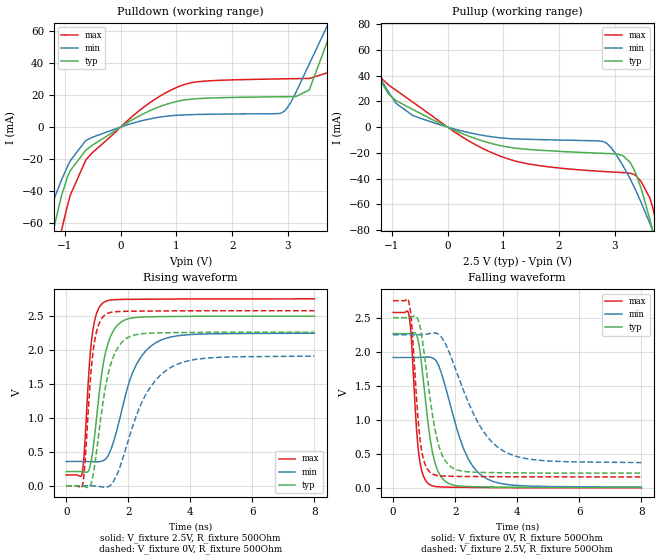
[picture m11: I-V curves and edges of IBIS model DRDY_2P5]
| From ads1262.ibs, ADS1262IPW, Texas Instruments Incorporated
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|   Model DRDY_2P5
[Model]   DRDY_2P5
Model_type   Output
Polarity   Non-Inverting
Enable   Active-Low
Vmeas = 1.25
Vref = 2.5
Cref = 15pF
Rref = 500
|   typ   min   max
|   (slow PVT)   (nom PVT)   (fast PVT)
C_comp   0.298p   0.274p   0.333p
|C_comp (ON state)   0.298p   0.282p   0.346p
|C_comp (OFF state)   0.298p   0.274p   0.333p
| Where   nom PVT is  Nominal Process, 2.5V, 27C
|   Fast PVT is Strong Process, 2.25V, -40C
|   Slow PVT is Weak Process, 2.75V, 125C
[Voltage Range]   2.5   2.25   2.75
[Temperature Range]   27   125   -40
[Pullup Reference]   2.5   2.25   2.75
[Pulldown Reference]   -0   -0   -0
[Power Clamp Reference]   2.5   2.25   2.75
[GND Clamp Reference]   -0   -0   -0
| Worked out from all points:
|   slope of the pulldown table from 0 to 0.375 V, typ, clamps not added: 48.4 ohm
|   slope of the pullup table from 0 to 0.375 V, typ, clamps not added: 54 ohm
|   falling waveform, V_fixture 0V, R_fixture 500Ohm: 20-80 % time 385ps typ, 813ps min, 219ps max; typ from 2.27 V to 0.006 V
|   rising waveform, V_fixture 2.5V, R_fixture 500Ohm: 20-80 % time 415ps typ, 791ps min, 236ps max; typ from 0.21 V to 2.5 V
|   rising waveform, V_fixture 0V, R_fixture 500Ohm: 20-80 % time 488ps typ, 1.03ns min, 262ps max; typ from 0 V to 2.26 V
|   falling waveform, V_fixture 2.5V, R_fixture 500Ohm: 20-80 % time 460ps typ, 1.13ns min, 251ps max; typ from 2.5 V to 0.216 V
[Pulldown]
|   Voltage   I(typ)   I(min)   I(max)
-2.5V     -315.8mA   -202.4mA   -454.5mA
-1.548V   -125.8mA   -82.52mA   -185.3mA
-1.315V   -83.24mA   -57.24mA   -122mA
-1.188V   -61.7mA    -44.53mA   -89.79mA
-1.06V    -42.72mA   -32.94mA   -64.38mA
-625mV    -14.46mA   -8.316mA   -20.61mA
950mV     15.58mA    7.244mA    24.01mA
2.877V    19mA       8.786mA    30.2mA
3.38V     23.15mA    39.24mA    30.47mA
3.703V    53.01mA    63.15mA    33.98mA
4.295V    106.5mA    98.71mA    106.7mA
4.992V    142.8mA    122.6mA    162.6mA
[Pullup]
|   Voltage   I(typ)   I(min)   I(max)
-2.5V     123.5mA    107.8mA    141.3mA
-1.87V    92.92mA    81.51mA    108.3mA
-1.645V   76.05mA    68.19mA    87.86mA
-1.06V    25.54mA    27.23mA    32.7mA
-625mV    13.67mA    9.005mA    19.41mA
950mV     -14.41mA   -8.361mA   -22.64mA
2.795V    -20.42mA   -11.34mA   -34.48mA
3.275V    -27.36mA   -40mA      -35.78mA
3.68V     -79.96mA   -80.27mA   -62.17mA
3.748V    -91.61mA   -87.8mA    -75.21mA
3.875V    -114.6mA   -102.5mA   -105.9mA
4.992V    -337mA     -247.2mA   -419.1mA
[Ramp]
R_load = 500
|   typ   min   max
dV/dt_r   1.3715/4.15054e-10   1.13197/7.90971e-10   1.55399/2.36049e-10
dV/dt_f   1.35577/3.84501e-10   1.14325/8.12774e-10   1.54566/2.19196e-10
[Falling Waveform]
V_fixture = 0V
V_fixture_min = 0V
V_fixture_max = 0V
R_fixture = 500Ohm
C_fixture = 0F
|   Time   V(typ)   V(min)   V(max)
0s        2.266V     1.915V     2.576V
504.3ps   2.265V     1.915V     2.549V
587.3ps   2.273V     1.915V     2.194V
817.8ps   2.142V     1.916V     535.8mV
943.9ps   1.704V     1.919V     217.6mV
1.18ns    768.1mV    1.919V     46.81mV
1.59ns    135.9mV    1.633V     12.85mV
2.278ns   22.4mV     565.7mV    7.372mV
2.883ns   14.06mV    171.6mV    5.396mV
8ns       5.923mV    9.605mV    126.9uV
[Rising Waveform]
V_fixture = 2.5V
V_fixture_min = 2.25V
V_fixture_max = 2.75V
R_fixture = 500Ohm
C_fixture = 0F
|   Time   V(typ)   V(min)   V(max)
0s        209.9mV    358.5mV    160mV
520.8ps   206.9mV    358.7mV    197.3mV
817.8ps   399.5mV    356mV      2.147V
943.9ps   855.7mV    353.9mV    2.485V
1.18ns    1.754V     369.1mV    2.69V
1.423ns   2.192V     517.1mV    2.732V
1.682ns   2.378V     907.7mV    2.74V
2.159ns   2.471V     1.687V     2.744V
2.883ns   2.488V     2.105V     2.746V
8ns       2.496V     2.245V     2.75V
[Rising Waveform]
V_fixture = 0V
V_fixture_min = 0V
V_fixture_max = 0V
R_fixture = 500Ohm
C_fixture = 0F
|   Time   V(typ)   V(min)   V(max)
0s        1.189nV    3.105nV    923.1pV
520.8ps   -2.675mV   352.2uV    4.909mV
859.8ps   145.8mV    -173.9uV   1.954V
1.038ns   726.6mV    -8.056mV   2.363V
1.257ns   1.435V     -19.06mV   2.518V
1.499ns   1.876V     49.57mV    2.557V
1.882ns   2.15V      492.2mV    2.566V
2.563ns   2.242V     1.342V     2.571V
3.363ns   2.252V     1.74V      2.573V
8ns       2.26V      1.907V     2.576V
[Falling Waveform]
|Gnd
V_fixture = 2.5V
V_fixture_min = 2.25V
V_fixture_max = 2.75V
R_fixture = 500Ohm
C_fixture = 0F
|   Time   V(typ)   V(min)   V(max)
0s        2.5V       2.25V      2.75V
504.3ps   2.499V     2.25V      2.739V
587.3ps   2.507V     2.25V      2.478V
901.9ps   2.288V     2.249V     594.3mV
1.257ns   1.109V     2.273V     205.3mV
1.499ns   579.5mV    2.243V     176.7mV
1.782ns   340.1mV    2.02V      171.2mV
2.723ns   228.6mV    969.8mV    165.9mV
3.523ns   222mV      550.2mV    163.3mV
8ns       216.4mV    371mV      160.1mV
